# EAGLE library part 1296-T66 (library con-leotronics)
1.27mm SINGLE ROW FEMALE SOCKET Source: http://www.leotronics.co.uk/Conexcon/Data%20Sheets/sec.%20A/1296ing.pdf
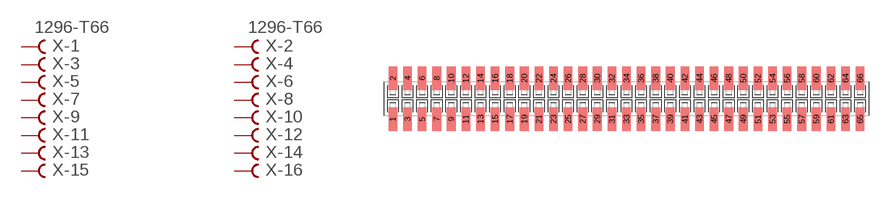
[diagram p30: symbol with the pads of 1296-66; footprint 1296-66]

Designator prefix X; gates -1=FVAL -2=FVAL -3=F -4=F -5=F -6=F -7=F -8=F -9=F -10=F -11=F -12=F -13=F -14=F -15=F -16=F -17=F -18=F -19=F -20=F -21=F -22=F -23=F -24=F -25=F -26=F -27=F -28=F -29=F -30=F -31=F -32=F -33=F -34=F -35=F -36=F -37=F -38=F -39=F -40=F -41=F -42=F -43=F -44=F -45=F -46=F -47=F -48=F -49=F -50=F -51=F -52=F -53=F -54=F -55=F -56=F -57=F -58=F -59=F -60=F -61=F -62=F -63=F -64=F -65=F -66=F

## 1296-T66 (OC_FARNELL: unknown; OC_NEWARK: unknown)  [1296-66]
1  -1:B  pas
2  -2:B  pas
3  -3:B  pas
4  -4:B  pas
5  -5:B  pas
6  -6:B  pas
7  -7:B  pas
8  -8:B  pas
9  -9:B  pas
10  -10:B  pas
11  -11:B  pas
12  -12:B  pas
13  -13:B  pas
14  -14:B  pas
15  -15:B  pas
16  -16:B  pas
17  -17:B  pas
18  -18:B  pas
19  -19:B  pas
20  -20:B  pas
21  -21:B  pas
22  -22:B  pas
23  -23:B  pas
24  -24:B  pas
25  -25:B  pas
26  -26:B  pas
27  -27:B  pas
28  -28:B  pas
29  -29:B  pas
30  -30:B  pas
31  -31:B  pas
32  -32:B  pas
33  -33:B  pas
34  -34:B  pas
35  -35:B  pas
36  -36:B  pas
37  -37:B  pas
38  -38:B  pas
39  -39:B  pas
40  -40:B  pas
41  -41:B  pas
42  -42:B  pas
43  -43:B  pas
44  -44:B  pas
45  -45:B  pas
46  -46:B  pas
47  -47:B  pas
48  -48:B  pas
49  -49:B  pas
50  -50:B  pas
51  -51:B  pas
52  -52:B  pas
53  -53:B  pas
54  -54:B  pas
55  -55:B  pas
56  -56:B  pas
57  -57:B  pas
58  -58:B  pas
59  -59:B  pas
60  -60:B  pas
61  -61:B  pas
62  -62:B  pas
63  -63:B  pas
64  -64:B  pas
65  -65:B  pas
66  -66:B  pas

## Footprint 1296-66 (pad centres in mm)
1.27mm SINGLE ROW FEMALE SOCKET Source: http://www.leotronics.co.uk/Conexcon/Data%20Sheets/sec.%20A/1296ing.pdf
smd 0.76 x 2.05: 1 -20.32,-1.78; 2 -20.32,1.78; 3 -19.05,-1.78; 4 -19.05,1.78; 5 -17.78,-1.78; 6 -17.78,1.78; 7 -16.51,-1.78; 8 -16.51,1.78; 9 -15.24,-1.78; 10 -15.24,1.78; 11 -13.97,-1.78; 12 -13.97,1.78; 13 -12.7,-1.78; 14 -12.7,1.78; 15 -11.43,-1.78; 16 -11.43,1.78; 17 -10.16,-1.78; 18 -10.16,1.78; 19 -8.89,-1.78; 20 -8.89,1.78; 21 -7.62,-1.78; 22 -7.62,1.78; 23 -6.35,-1.78; 24 -6.35,1.78; 25 -5.08,-1.78; 26 -5.08,1.78; 27 -3.81,-1.78; 28 -3.81,1.78; 29 -2.54,-1.78; 30 -2.54,1.78; 31 -1.27,-1.78; 32 -1.27,1.78; 33 0,-1.78; 34 0,1.78; 35 1.27,-1.78; 36 1.27,1.78; 37 2.54,-1.78; 38 2.54,1.78; 39 3.81,-1.78; 40 3.81,1.78; 41 5.08,-1.78; 42 5.08,1.78; 43 6.35,-1.78; 44 6.35,1.78; 45 7.62,-1.78; 46 7.62,1.78; 47 8.89,-1.78; 48 8.89,1.78; 49 10.16,-1.78; 50 10.16,1.78; 51 11.43,-1.78; 52 11.43,1.78; 53 12.7,-1.78; 54 12.7,1.78; 55 13.97,-1.78; 56 13.97,1.78; 57 15.24,-1.78; 58 15.24,1.78; 59 16.51,-1.78; 60 16.51,1.78; 61 17.78,-1.78; 62 17.78,1.78; 63 19.05,-1.78; 64 19.05,1.78; 65 20.32,-1.78; 66 20.32,1.78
